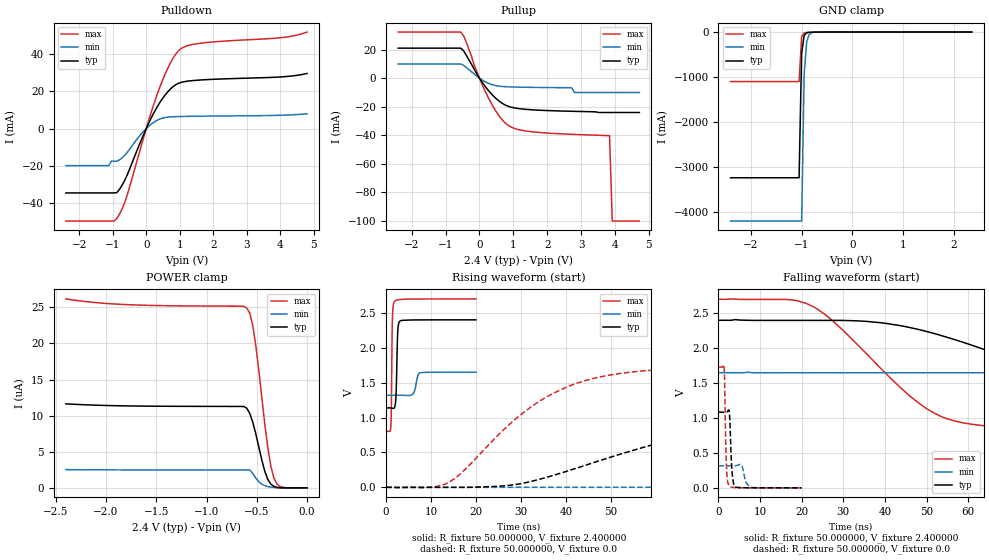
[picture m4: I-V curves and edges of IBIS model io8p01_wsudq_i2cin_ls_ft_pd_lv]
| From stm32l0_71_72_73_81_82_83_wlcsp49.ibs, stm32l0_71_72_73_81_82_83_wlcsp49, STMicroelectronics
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|   Model io8p01_wsudq_i2cin_ls_ft_pd_lv
[Model]  io8p01_wsudq_i2cin_ls_ft_pd_lv
Model_type I/O
Polarity   Non-Inverting
Enable   Active-Low
Vinl =   0.720000V
Vinh =   1.680000V
Vmeas =  1.200000V
Cref =   50.000000pF
Rref =   100.000000M
Vref =   0.0V
C_comp   2.943600pF   2.919700pF   2.965100pF
[Temperature Range]   25.000000   0.105000k   -40.000000
[Pullup Reference]   2.400000V   1.650000V   2.700000V
[Pulldown Reference]   0.0V   0.0V   0.0V
[POWER Clamp Reference]   2.400000V   1.650000V   2.700000V
[GND Clamp Reference]   0.0V   0.0V   0.0V
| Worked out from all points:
|   slope of the pulldown table from 0 to 0.36 V, typ, clamps not added: 28.5 ohm
|   slope of the pullup table from 0 to 0.36 V, typ, clamps not added: 32.2 ohm
|   GND clamp passes 1 mA (typ) near -0.64 V on its own axis
|   rising waveform, R_fixture 50.000000, V_fixture 2.400000: 20-80 % time 285ps typ, 639ps min, 195ps max; typ from 1.14 V to 2.4 V
|   rising waveform, R_fixture 50.000000, V_fixture 0.0: 20-80 % time 39.7ns typ, 106ns min, 19.4ns max; typ from 0 V to 1.08 V
|   falling waveform, R_fixture 50.000000, V_fixture 2.400000: 20-80 % time 40.8ns typ, 106ns min, 20.1ns max; typ from 2.4 V to 1.14 V
|   falling waveform, R_fixture 50.000000, V_fixture 0.0: 20-80 % time 482ps typ, 851ps min, 380ps max; typ from 1.08 V to 0 V
[Pulldown]
|Voltage   I(typ)   I(min)   I(max)
-2.4V     -34.7mA    -20mA      -49.82mA
-1.12V    -34.7mA    -20mA      -49.82mA
-1.04V    -34.7mA    -17.6mA    -49.82mA
-880mV    -34.55mA   -17.6mA    -48.46mA
-560mV    -24.65mA   -12.68mA   -35.33mA
0V        326fA      0A         140fA
400mV     13.84mA    5.066mA    22.03mA
720mV     21.25mA    6.254mA    35.26mA
1.04V     24.83mA    6.464mA    43.03mA
1.6V      26.11mA    6.627mA    45.88mA
4V        27.76mA    7.125mA    48.88mA
4.8V      29.63mA    7.94mA     51.96mA
[Pullup]
|Voltage   I(typ)   I(min)   I(max)
-2.4V     21.06mA    9.988mA    32.35mA
-560mV    21.06mA    9.988mA    32.35mA
-400mV    16.53mA    7.734mA    25.89mA
-80mV     3.011mA    1.498mA    4.671mA
320mV     -10.16mA   -4.078mA   -16.34mA
640mV     -17.08mA   -5.718mA   -28.28mA
960mV     -20.45mA   -6.129mA   -34.5mA
1.76V     -22.39mA   -6.471mA   -37.97mA
2.8V      -23.2mA    -10mA      -39.35mA
3.84V     -24mA      -10mA      -40.2mA
3.92V     -24mA      -10mA      -100mA
4.72V     -24mA      -10mA      -100mA
[GND_clamp]
|Voltage   I(typ)   I(min)   I(max)
-2.4V     -3.237A    -4.198A    -1.1A
-1.05V    -3.237A    -4.198A    -1.1A
-1V       -475.8mA   -4.198A    -104.2mA
-950mV    -76.26mA   -935.5mA   -18.4mA
-900mV    -16.62mA   -212.9mA   -9.114mA
-850mV    -6.559mA   -50.96mA   -6.598mA
-800mV    -4.01mA    -13.82mA   -4.868mA
-650mV    -1.055mA   -1.198mA   -1.154mA
2.35V     52.69uA    50.02uA    36.84uA
[POWER_clamp]
|Voltage   I(typ)   I(min)   I(max)
-2.4V     11.64uA    2.525uA    26.17uA
-1.86V    11.37uA    2.488uA    25.42uA
-600mV    11.04uA    2.474uA    24.9uA
-570mV    10.3uA     2.473uA    24.21uA
-540mV    9.097uA    2uA        22.48uA
-510mV    7.497uA    1.35uA     19.73uA
-450mV    3.845uA    512.5nA    12.52uA
-390mV    1.154uA    175.5nA    5.528uA
-360mV    508.2nA    102.8nA    2.997uA
-330mV    204.4nA    60.39nA    1.375uA
-270mV    0A         0A         194.9nA
0V        0A         0A         0A
[Ramp]
| variable   typ   min   max
dV/dt_r  0.65010/39.65154n   0.18951/0.10641u   1.03746/19.39045n
dV/dt_f  0.75702/40.77563n   0.19512/0.10564u   1.13800/20.06866n
R_load = 50.000000
[Rising Waveform]
R_fixture= 50.000000
V_fixture= 2.400000
V_fixture_min= 1.650000
V_fixture_max= 2.700000
|time   V(typ)   V(min)   V(max)
0s        1.137V     1.32V      802.9mV
1.041ns   1.137V     1.32V      868mV
1.161ns   1.136V     1.32V      1.176V
1.401ns   1.132V     1.32V      2.435V
1.842ns   1.142V     1.32V      2.662V
2.202ns   1.334V     1.32V      2.679V
2.603ns   2.258V     1.32V      2.685V
3.003ns   2.377V     1.32V      2.689V
7.648ns   2.398V     1.641V     2.697V
19.94ns   2.399V     1.649V     2.7V
[Rising Waveform]
R_fixture= 50.000000
V_fixture= 0.0
V_fixture_min= 0.0
V_fixture_max= 0.0
|time   V(typ)   V(min)   V(max)
0s        1.509nV    7.645nV    1.259nV
14.01ns   -216.4uV   -47.28uV   76.05mV
30.03ns   54.33mV    -45.93uV   1.047V
40.04ns   228.6mV    -45.77uV   1.435V
49.05ns   415.3mV    -42.33uV   1.601V
63.06ns   671.4mV    34.57uV    1.694V
86.09ns   924mV      1.081mV    1.725V
125.1ns   1.058V     43.42mV    1.729V
255.3ns   1.084V     267mV      1.729V
498.5ns   1.083V     316.1mV    1.729V
[Falling Waveform]
R_fixture= 50.000000
V_fixture= 2.400000
V_fixture_min= 1.650000
V_fixture_max= 2.700000
|time   V(typ)   V(min)   V(max)
0s        2.399V     1.649V     2.7V
21.02ns   2.397V     1.648V     2.642V
28.03ns   2.397V     1.648V     2.36V
50.05ns   2.238V     1.648V     1.133V
57.06ns   2.116V     1.648V     952.9mV
69.07ns   1.869V     1.648V     863.6mV
99.1ns    1.361V     1.647V     814.9mV
144.1ns   1.186V     1.626V     804.1mV
286.3ns   1.138V     1.38V      802.9mV
498.5ns   1.137V     1.32V      802.9mV
[Falling Waveform]
R_fixture= 50.000000
V_fixture= 0.0
V_fixture_min= 0.0
V_fixture_max= 0.0
|time   V(typ)   V(min)   V(max)
0s        1.083V     316.1mV    1.729V
1.361ns   1.083V     316.1mV    1.719V
1.882ns   1.083V     316.1mV    364.7mV
2.122ns   1.09V      316.1mV    124.8mV
2.523ns   1.11V      316.1mV    32.25mV
3.243ns   241.3mV    315.9mV    7.623mV
4.004ns   16.96mV    316.2mV    3.967mV
5.566ns   2.082mV    322.1mV    1.856mV
7.968ns   878.7uV    8.135mV    706.6uV
19.94ns   1.509nV    7.645nV    1.259nV
